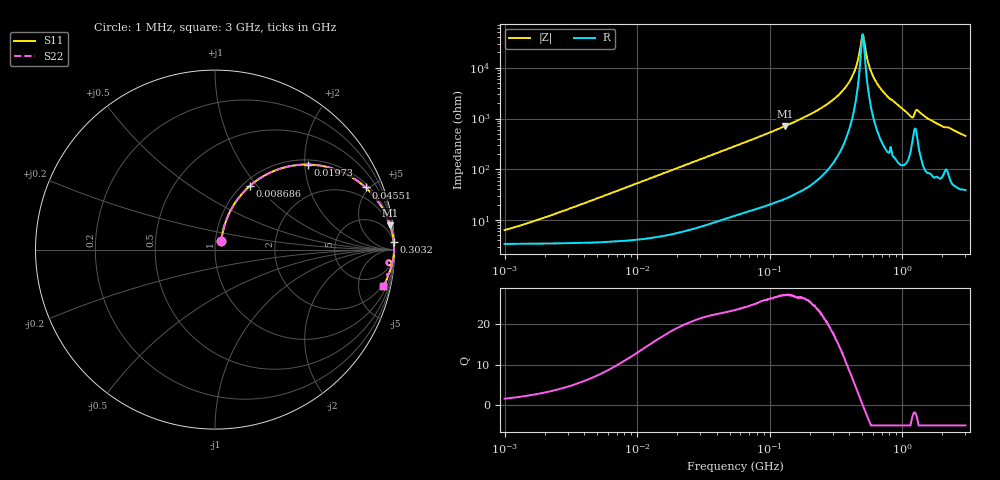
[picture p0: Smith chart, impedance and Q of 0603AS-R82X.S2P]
!s-Parameter Generated by FASTRON Sdn. Bhd.
!FASTRON P/N : 0603AS-R82X
!Keysight Technologies: E4991B_MY54100416_A.01.15
!Date created: Tue Oct 17 15:26:42 2023
!Version  : Rev01 Tue Oct 17 15:26:42 2023
!Data & Calibration Information:
!Freq	S11	S21	S12	S22
!PortZ  Port1:50+j0  Port2:50+j0
!When reading reference impedance value at option line is always used.
! Remarks : This data is being provided solely for informational purposes.
# Hz S dB R 50
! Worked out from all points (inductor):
!   1601 points, 1 MHz to 3 GHz, reference 50 ohm
!   read as one part in series: L = 847 nH near 1.946 MHz
!   highest Q = 27.1 at 131.5 MHz (marker M1), where L = 862 nH
!   self-resonance near 502.7 MHz
!   S11 on the Smith chart (normalised r, x): 1 MHz: 1.07, +0.11; 8.686 MHz: 1.08, +0.92; 19.73 MHz: 1.11, +2.07; 45.51 MHz: 1.21, +4.74; 303.2 MHz: 4, +47; 3 GHz: 1.78, -9.02
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1000000  -24.26 54.7  -0.30 -3.0  -0.30 -3.0  -24.26 54.7
3804036  -14.23 69.0  -0.46 -11.0  -0.46 -11.0  -14.23 69.0
8686058  -7.84 61.3  -1.11 -23.8  -1.11 -23.8  -7.84 61.3
1.447069e7  -4.59 50.4  -2.24 -36.1  -2.24 -36.1  -4.59 50.4
1.973457e7  -3.07 42.5  -3.40 -44.5  -3.40 -44.5  -3.07 42.5
4.551475e7  -0.84 22.4  -8.35 -65.0  -8.35 -65.0  -0.84 22.4
5.477226e7  -0.62 19.0  -9.73 -68.5  -9.73 -68.5  -0.62 19.0
1.314834e8  -0.13 7.9  -17.19 -79.9  -17.19 -79.9  -0.13 7.9
2.083556e8  -0.05 4.5  -22.07 -83.2  -22.07 -83.2  -0.05 4.5
3.032461e8  -0.03 2.4  -27.53 -84.3  -27.53 -84.3  -0.03 2.4
4.177151e8  -0.02 0.9  -36.36 -80.9  -36.36 -80.9  -0.02 0.9
4.525341e8  -0.02 0.5  -40.99 -75.3  -40.99 -75.3  -0.02 0.5
4.902556e8  -0.02 0.1  -50.08 -45.7  -50.08 -45.7  -0.02 0.1
5.026765e8  -0.02 0.0  -53.12 -5.7  -53.12 -5.7  -0.02 0.0
5.154121e8  -0.02 -0.1  -50.95 38.2  -50.95 38.2  -0.02 -0.1
5.555877e8  -0.02 -0.4  -41.84 73.2  -41.84 73.2  -0.02 -0.4
6.018993e8  -0.02 -0.8  -36.79 79.8  -36.79 79.8  -0.02 -0.8
7.925923e8  -0.03 -2.2  -28.19 83.0  -28.19 83.0  -0.03 -2.2
1.159346e9  -0.20 -5.0  -21.01 73.1  -21.01 73.1  -0.20 -5.0
1.313842e9  -0.16 -3.8  -23.31 72.4  -23.31 72.4  -0.16 -3.8
1.773925e9  -0.15 -6.8  -18.53 78.4  -18.53 78.4  -0.15 -6.8
3e9  -0.36 -12.2  -13.47 72.9  -13.47 72.9  -0.36 -12.2
